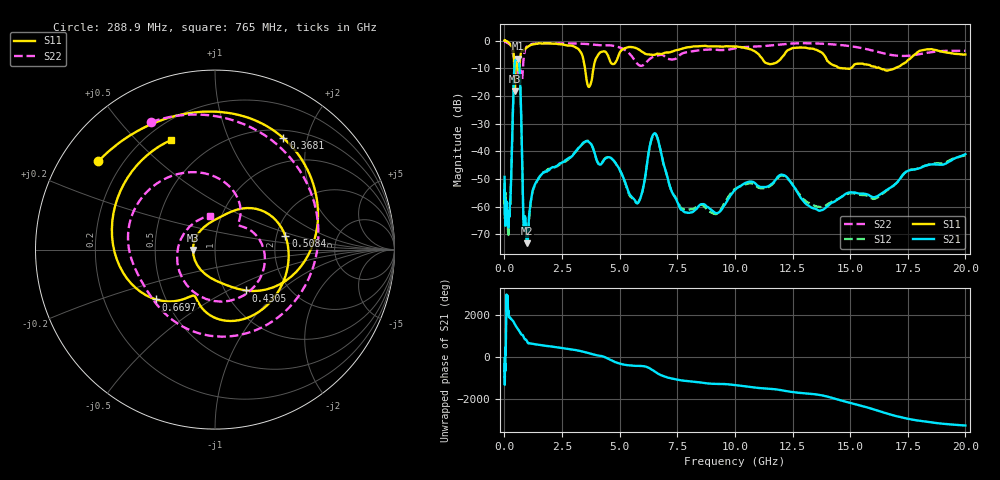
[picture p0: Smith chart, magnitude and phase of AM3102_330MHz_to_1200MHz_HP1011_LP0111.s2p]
! Date/Time: Tue, Sep 11, 2018 5:20 PM
! Network Analyzer: Agilent Technologies E8362B Rev: A.07.50.63
! Sweep from 0.010 to 20.000 GHz, 1601 Points, Sweep Type: LOG
! Power Supply: 4.949 V, 0.001 A
# Hz S DB R 50
!freq MagS11 AngS11 MagS21 AngS21 MagS12 AngS12 MagS22 AngS22
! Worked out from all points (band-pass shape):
!   1601 points, 10 MHz to 20 GHz, reference 50 ohm
!   highest |S21| = -6.52 dB at 589.1 MHz (marker M1); lowest = -73.3 dB at 993.4 MHz (marker M2)
!   |S21| within 3 dB of the highest: 435 MHz to 651.8 MHz (216.8 MHz wide, 39.9 % of centre)
!   lowest |S11| = -18.2 dB at 453.6 MHz (marker M3), VSWR 1.28, Z = 39.1 - j0.14 ohm
!   |S11| at or under -10 dB: 3.498 GHz to 3.865 GHz (366.6 MHz wide, 9.96 % of centre); 14.64 GHz to 15.03 GHz (388.5 MHz wide, 2.62 % of centre); 16.29 GHz to 16.95 GHz (659 MHz wide, 3.96 % of centre)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
!   |S22| runs from -14.5 to -0.1 dB; largest |S21 - S12| = 0.0086
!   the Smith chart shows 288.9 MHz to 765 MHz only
!   S11 on the Smith chart (normalised r, x): 288.9 MHz: 0.11, +0.33; 368.1 MHz: 0.61, +1.62; 430.5 MHz: 1.24, -0.61; 508.4 MHz: 2.24, +0.40; 669.7 MHz: 0.44, -0.30; 765 MHz: 0.30, +0.63
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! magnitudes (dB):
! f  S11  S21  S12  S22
! 10 MHz  0.0  -49.3  -56.6  -0.1
! 35.55 MHz  0.0  -62.4  -64.6  -0.4
! 126.4 MHz  -0.4  -64.6  -64.1  -0.9
! 288.9 MHz  -1.8  -51.3  -51.6  -2.0
! 368.1 MHz  -2.8  -25.9  -25.9  -4.6
! 430.5 MHz  -10.9  -10.1  -10.2  -6.8
! 447.2 MHz  -17.6  -8.2  -8.3  -7.1
! 453.6 MHz  -18.2  -7.8  -7.8  -7.1
! 508.4 MHz  -8.0  -7.0  -7.0  -6.0
! 589.1 MHz  -8.9  -6.5  -6.7  -10.1
! 669.7 MHz  -7.3  -12.1  -12.1  -11.6
! 765 MHz  -3.6  -40.4  -40.5  -14.4
! 837.2 MHz  -3.4  -67.0  -67.0  -6.3
! 993.4 MHz  -2.4  -73.3  -74.2  -1.9
! 1.59 GHz  -1.1  -48.5  -48.5  -1.0
! 3.617 GHz  -16.1  -36.4  -36.2  -1.3
! 5.652 GHz  -2.5  -57.6  -57.9  -7.1
! 6.518 GHz  -5.1  -33.5  -33.7  -5.7
! 7.958 GHz  -2.4  -62.3  -61.1  -4.1
! 11.97 GHz  -6.8  -48.5  -48.9  -1.4
! 13.81 GHz  -4.6  -61.2  -60.2  -1.2
! 20 GHz  -5.0  -41.1  -41.5  -3.7
